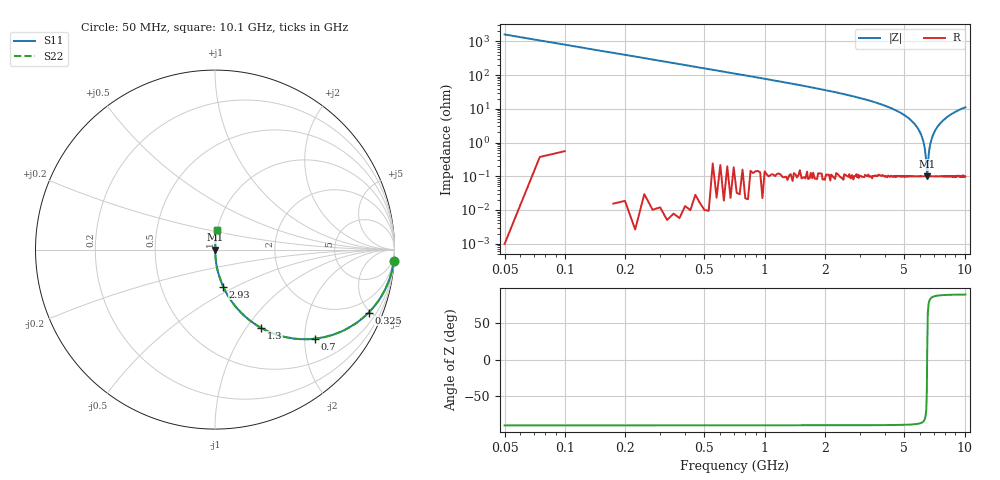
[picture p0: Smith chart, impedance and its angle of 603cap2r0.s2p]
! AVX Thin Film Operation		Date: November 2004
! Description: Accu-P® Series, Thin Film, SMD, RF Capacitor
! Part Number: 06035J2R0ABT
! 50 MHz  -  10.05 GHz
! Serial Measurements
# hz S db R 50
!	S11		S21		S12		S22
!	dB	Phase	dB	Phase	dB	Phase	dB	Phase
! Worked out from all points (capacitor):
!   400 points, 50 MHz to 10.1 GHz, reference 50 ohm
!   read as one part in series: C = 2 pF near 100 MHz
!   lowest |Z| = 100 mohm at 6.5 GHz (marker M1)
!   series resonance near 6.498 GHz, so ESL is about 300 pH
!   S11 on the Smith chart (normalised r, x): 50 MHz: 1, -32; 325 MHz: 1.00, -4.88; 700 MHz: 1.00, -2.25; 1.3 GHz: 1.00, -1.18; 2.93 GHz: 1.00, -0.43; 10.1 GHz: 1.00, +0.22
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5e7  -0.02 -3.6  -24.10 86.4  -24.10 86.4  -0.02 -3.6
1e8  -0.07 -7.2  -18.10 82.8  -18.10 82.8  -0.07 -7.2
1.5e8  -0.15 -10.7  -14.60 79.3  -14.60 79.3  -0.15 -10.7
3.25e8  -0.67 -22.3  -8.43 67.7  -8.43 67.7  -0.67 -22.3
7e8  -2.54 -41.6  -3.55 48.3  -3.55 48.3  -2.54 -41.6
1.3e9  -5.91 -59.5  -1.29 30.4  -1.29 30.4  -5.91 -59.5
1.73e9  -8.10 -66.7  -0.74 23.2  -0.74 23.2  -8.10 -66.7
2.93e9  -13.50 -77.5  -0.21 12.2  -0.21 12.2  -13.50 -77.5
3.4e9  -15.50 -80.0  -0.13 9.6  -0.13 9.6  -15.50 -80.0
5.08e9  -24.30 -85.6  -0.02 3.5  -0.02 3.5  -24.30 -85.6
5.63e9  -29.00 -86.4  -0.01 2.0  -0.01 2.0  -29.00 -86.4
6.13e9  -36.80 -85.2  -0.01 0.8  -0.01 0.8  -36.80 -85.2
6.28e9  -41.30 -82.8  -0.01 0.5  -0.01 0.5  -41.30 -82.8
6.38e9  -46.40 -77.6  -0.01 0.3  -0.01 0.3  -46.40 -77.6
6.43e9  -50.70 -69.8  -0.01 0.2  -0.01 0.2  -50.70 -69.8
6.5e9  -60.00 5.4  -0.01 -0.0  -0.01 -0.0  -60.00 5.4
6.6e9  -48.00 75.2  -0.01 -0.2  -0.01 -0.2  -48.00 75.2
6.75e9  -40.60 83.4  -0.01 -0.5  -0.01 -0.5  -40.60 83.4
6.95e9  -35.60 85.6  -0.01 -0.9  -0.01 -0.9  -35.60 85.6
7.4e9  -29.90 86.4  -0.01 -1.8  -0.01 -1.8  -29.90 86.4
8.43e9  -23.90 85.4  -0.03 -3.7  -0.03 -3.7  -23.90 85.4
1.01e10  -19.20 83.2  -0.06 -6.3  -0.06 -6.3  -19.20 83.2
